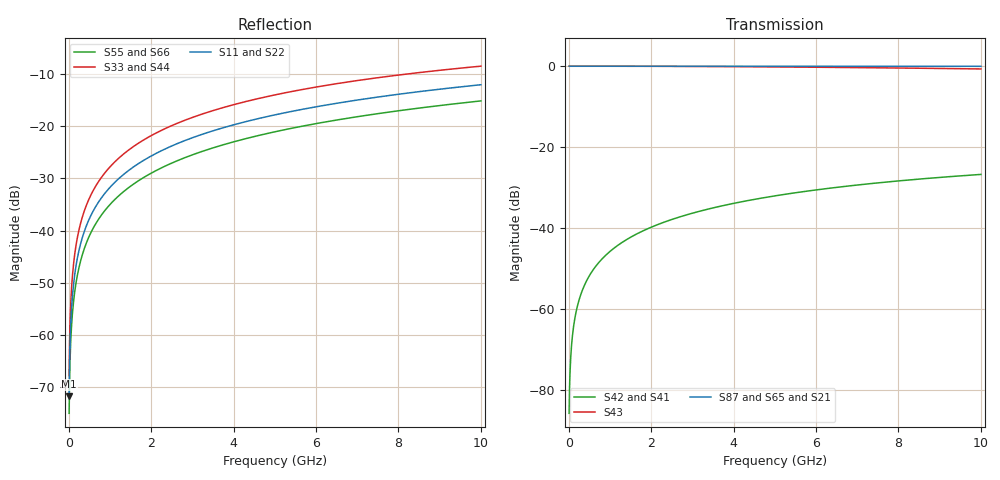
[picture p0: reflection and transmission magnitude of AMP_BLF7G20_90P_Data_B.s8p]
! Created Tue May 08 14:05:32 2012
# ghz S ma R 50
! 8 Port Network Data from SP1.SP block
! freq  magS11  angS11  magS12  angS12  magS13  angS13  magS14  angS14
!  magS15  angS15  magS16  angS16  magS17  angS17  magS18  angS18
!  magS21  angS21  magS22  angS22  magS23  angS23  magS24  angS24
!  magS25  angS25  magS26  angS26  magS27  angS27  magS28  angS28
!  magS31  angS31  magS32  angS32  magS33  angS33  magS34  angS34
!  magS35  angS35  magS36  angS36  magS37  angS37  magS38  angS38
!  magS41  angS41  magS42  angS42  magS43  angS43  magS44  angS44
!  magS45  angS45  magS46  angS46  magS47  angS47  magS48  angS48
!  magS51  angS51  magS52  angS52  magS53  angS53  magS54  angS54
!  magS55  angS55  magS56  angS56  magS57  angS57  magS58  angS58
!  magS61  angS61  magS62  angS62  magS63  angS63  magS64  angS64
!  magS65  angS65  magS66  angS66  magS67  angS67  magS68  angS68
!  magS71  angS71  magS72  angS72  magS73  angS73  magS74  angS74
!  magS75  angS75  magS76  angS76  magS77  angS77  magS78  angS78
!  magS81  angS81  magS82  angS82  magS83  angS83  magS84  angS84
!  magS85  angS85  magS86  angS86  magS87  angS87  magS88  angS88
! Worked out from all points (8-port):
!   1000 points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, 10 MHz to 10 GHz, reference 50 ohm
!   strongest paths, dB at 10 MHz, 2.51 GHz, 5.01 GHz, 7.51 GHz, 10 GHz:
!     S87: 0.0, 0.0, 0.0, 0.0, 0.0
!     S65: 0.0, 0.0, 0.0, -0.1, -0.1
!     S21: 0.0, 0.0, -0.1, -0.2, -0.3
!     S43: 0.0, 0.0, -0.2, -0.4, -0.7
!     S42: -85.8, -37.8, -32.0, -28.8, -26.7
!     S41: -85.8, -37.8, -32.0, -28.8, -26.7
!   lowest |S11| = -71.7 dB at 10 MHz (marker M1), VSWR 1.00, Z = 50 + j0.0259 ohm
!   |S11| at or under -10 dB: start of sweep to end of sweep
